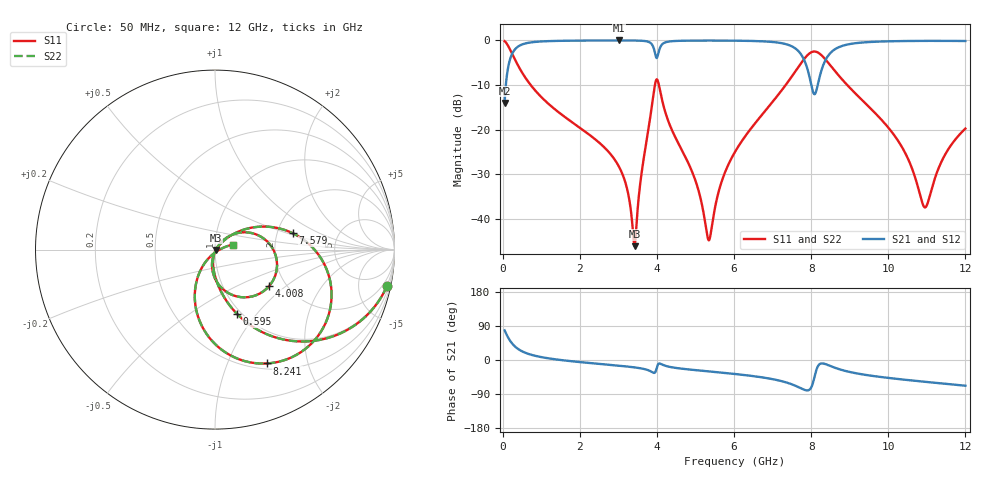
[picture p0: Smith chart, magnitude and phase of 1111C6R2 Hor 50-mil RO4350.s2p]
# GHz S MA R 50
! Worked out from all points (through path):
!   11951 points, 50 MHz to 12 GHz, reference 50 ohm
!   highest |S21| = -0.03 dB at 3.019 GHz (marker M1); lowest = -14.0 dB at 50 MHz (marker M2)
!   group delay of S21, straight-line fit = 18 ps
!   lowest |S11| = -46.0 dB at 3.42 GHz (marker M3), VSWR 1.01, Z = 50.5 - j0.22 ohm
!   |S11| at or under -10 dB: 727 MHz to 3.948 GHz (3.221 GHz wide, 138 % of centre); 4.052 GHz to 7.339 GHz (3.287 GHz wide, 57.7 % of centre); 8.936 GHz to end of sweep
!   |S22| runs from -46.0 to -0.2 dB; largest |S21 - S12| = 0
!   S11 on the Smith chart (normalised r, x): 50 MHz: 0.95, -9.59; 595 MHz: 0.95, -0.80; 4.008 GHz: 1.64, -0.77; 7.579 GHz: 2.44, +0.55; 8.241 GHz: 0.57, -1.40; 12 GHz: 1.22, +0.07
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0.05  0.9799 -11.8  0.1994 78.2  0.1994 78.2  0.9799 -11.8
0.23  0.7295 -44.5  0.6836 45.5  0.6836 45.5  0.7295 -44.5
0.595  0.3787 -71.1  0.9248 18.8  0.9248 18.8  0.3787 -71.1
2.042  0.1022 -95.2  0.9934 -5.9  0.9934 -5.9  0.1022 -95.2
3.019  0.03846 -101.7  0.9968 -15.1  0.9968 -15.1  0.03846 -101.7
3.234  0.02118 -98.7  0.9964 -17.3  0.9964 -17.3  0.02118 -98.7
3.42  0.004997 -25.9  0.9948 -19.5  0.9948 -19.5  0.004997 -25.9
3.875  0.1922 30.1  0.895 -31.9  0.895 -31.9  0.1922 30.1
4.008  0.3637 -34.1  0.6471 -16.5  0.6471 -16.5  0.3637 -34.1
4.034  0.3399 -48.9  0.7098 -10.9  0.7098 -10.9  0.3399 -48.9
4.249  0.1423 -93.0  0.9576 -16.2  0.9576 -16.2  0.1423 -93.0
4.993  0.02749 -103.1  0.9929 -26.7  0.9929 -26.7  0.02749 -103.1
5.337  0.005851 -36.4  0.9939 -30.0  0.9939 -30.0  0.005851 -36.4
6.025  0.05658 46.0  0.9911 -36.9  0.9911 -36.9  0.05658 46.0
7.579  0.4424 11.9  0.8185 -67.4  0.8185 -67.4  0.4424 11.9
8.017  0.7401 -33.9  0.2994 -69.1  0.2994 -69.1  0.7401 -33.9
8.241  0.6979 -65.3  0.4226 -9.7  0.4226 -9.7  0.6979 -65.3
8.723  0.4003 -102.8  0.8405 -24.1  0.8405 -24.1  0.4003 -102.8
10.009  0.1047 -127.0  0.9753 -47.4  0.9753 -47.4  0.1047 -127.0
10.953  0.01353 -55.8  0.9859 -57.5  0.9859 -57.5  0.01353 -55.8
11.437  0.04934 13.1  0.9859 -62.4  0.9859 -62.4  0.04934 13.1
12  0.1031 15.6  0.9825 -67.9  0.9825 -67.9  0.1031 15.6
